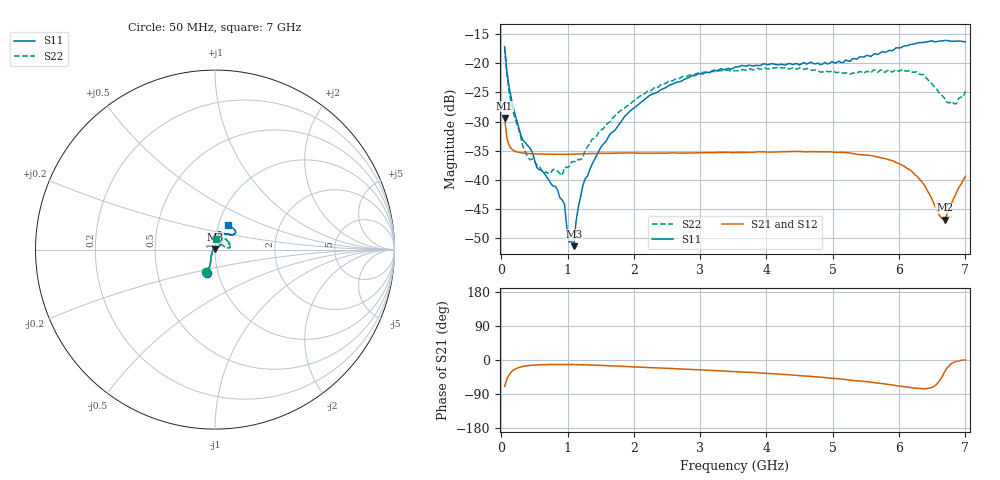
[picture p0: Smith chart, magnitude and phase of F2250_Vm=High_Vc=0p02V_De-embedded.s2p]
! Integrated Device Technology
! Corporate Headquarters
! 6024 Silver Creek Valley Road
! San Jose, CA 95138  USA
! Phone:  1-408-284-8200
! Toll Free:  1-800-223-1366
! Webpage:  http://www.idt.com/
! Timing and RF Division
! 515 Groton Road, Suite 102
! Westford, MA 01886-6024
! Device:  F2250
! Description: Voltage Variable RF Attenuator
! Frequency:  50.0 -  6000.00 MHz
! Package:  3x3 mm Thin QFN Plastic Package: 16 pin
! Ports:  2 RF, 3 DC
!  Pin  1  = GND
!  Pin  2  = NC
!  Pin  3  = RF1  = Port 1
!  Pin  4  = NC
!  Pin  5  = GND
!  Pin  6  = GND
!  Pin  7  = GND
!  Pin  8  = GND
!  Pin  9  = NC
!  Pin 10  = RF2  = Port 2
!  Pin 11  = NC
!  Pin 12  = GND
!  Pin 13  = GND
!  Pin 14  = VCNTRL
!  Pin 15  = VDD
!  Pin 16  = VMODE
! Vcntrl:  0.020 Volts
! Vmode:  +3.300 Volts
! Vdd:  +3.30  Volts
! Current:  1.244 mA
! Data:  The device was measured on a the F2250 evaluation board which has
!  individual transmission lines to the RF pins.  Data was collected
!  using a calibrated network analyzer.  The evaluation board was
!  de-embedded using a TRL calibration technique.
!  The reference plane is the edge of the package pin.
! Misc:  SN 10
!  Action Tracker AT0258
! Date Measured:  2014-11-26
! Date:  2015-10-15  MJV
! Note:
!  Integrated Device Technology supplies this data as a sample of measured
!  data at the package pin for this product.  Your particular data for this
!  product may vary.
!  Data was taken at 25 degrees C.
!  Integrated Device Technology reserves the right to change this data at anytime.
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# GHz S dB R 50
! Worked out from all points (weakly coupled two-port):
!   201 points, 50 MHz to 7 GHz, reference 50 ohm
!   highest |S21| = -29.38 dB at 50 MHz (marker M1); lowest = -46.8 dB at 6.687 GHz (marker M2)
!   lowest |S11| = -51.4 dB at 1.093 GHz (marker M3), VSWR 1.01, Z = 50 + j0.27 ohm
!   |S11| at or under -10 dB: start of sweep to end of sweep
!   |S22| runs from -39.2 to -17.4 dB; largest |S21 - S12| = 6.3e-05
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0.05  -17.18 -108.5  -29.38 -69.5  -29.38 -69.5  -17.37 -110.6
0.08475  -21.47 -107.4  -32.86 -50.1  -32.86 -50.1  -21.87 -109.0
0.15425  -26.22 -116.6  -34.68 -31.0  -34.68 -31.0  -27.10 -120.7
0.29325  -32.27 -127.5  -35.35 -18.5  -35.35 -18.4  -32.66 -133.6
0.3975  -34.11 -142.2  -35.48 -15.0  -35.48 -15.1  -36.09 -158.3
0.5365  -37.88 -154.7  -35.55 -12.9  -35.55 -12.9  -37.49 180.0
0.64075  -38.77 -162.7  -35.58 -12.2  -35.58 -12.2  -38.88 160.5
0.91875  -43.45 156.0  -35.60 -11.8  -35.60 -11.8  -39.23 128.0
0.9535  -44.20 170.7  -35.60 -11.8  -35.60 -11.8  -37.82 124.2
1.023  -50.67 140.9  -35.59 -11.9  -35.59 -11.9  -37.71 108.1
1.0925  -51.36 89.3  -35.57 -12.0  -35.58 -12.0  -36.84 98.8
1.12725  -47.14 61.7  -35.57 -12.1  -35.56 -12.1  -36.91 91.7
1.2315  -40.87 40.5  -35.52 -12.5  -35.53 -12.5  -36.06 77.3
1.6485  -32.03 41.2  -35.44 -15.2  -35.44 -15.2  -29.92 60.0
2.37825  -24.76 46.7  -35.40 -21.0  -35.40 -21.0  -24.03 53.9
3.525  -20.66 71.7  -35.32 -30.6  -35.32 -30.6  -21.26 73.0
4.7065  -20.06 72.0  -35.15 -43.9  -35.16 -43.9  -21.21 70.4
5.85325  -17.79 40.5  -36.57 -64.8  -36.58 -64.9  -21.13 23.4
6.27025  -16.53 39.4  -39.40 -74.5  -39.40 -74.6  -21.46 8.6
6.68725  -16.11 47.9  -46.81 -31.0  -46.78 -30.6  -26.02 28.5
6.861  -16.21 54.5  -42.30 -3.7  -42.26 -3.8  -26.96 57.4
7  -16.32 62.5  -39.36 -0.1  -39.33 -0.3  -24.82 83.6
